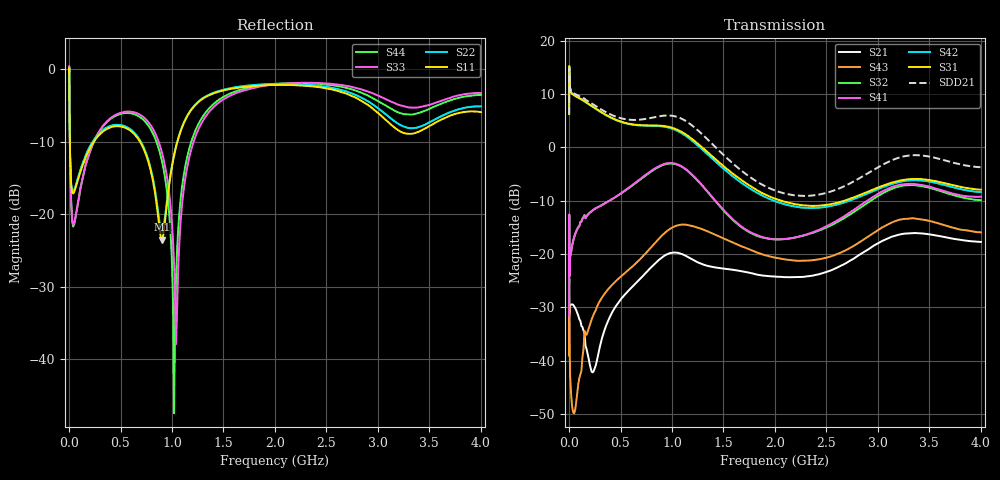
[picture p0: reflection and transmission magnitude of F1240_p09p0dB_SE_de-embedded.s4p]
! Integrated Device Technology
! Corporate Headquarters
! 6024 Silver Creek Valley Road
! San Jose, CA 95138  USA
! Phone:  1-408-284-8200
! Toll Free:  1-800-223-1366
! Webpage:  http://www.idt.com/
! Timing and RF Division
! 515 Groton Road, Suite 102
! Westford, MA 01886-6024
! Device:  F1240
! Description: Dual Intermediate Frequency Digital Variable Gain Amplifier
! Frequency:  10.0 -  500.00 MHz
! Package:  5x5 mm QFN Plastic Package: 32 pin
! Ports:  8 RF, 20 DC
!  Pin  1  = GA3 / Data  Pin 17  = RF OUT_B+
!  Pin  2  = GA4 / CLK  Pin 18  = RF OUT_B-
!  Pin  3  = GA5  Pin 19  = STBY_B
!  Pin  4  = VMODE  Pin 20  = Ground
!  Pin  5  = No Connect  Pin 21  = Ground
!  Pin  6  = GB5  Pin 22  = STB_A
!  Pin  7  = GB4  Pin 23  = RF OUT_A-  = Port 4
!  Pin  8  = GB3  Pin 24  = RF OUT_A+  = Port 3
!  Pin  9  = GB2  Pin 25  = GA0
!  Pin 10  = GB1  Pin 26  = ISET_A
!  Pin 11  = RF IN_B+  Pin 27  = VCC
!  Pin 12  = RF IN_B-  Pin 28  = Ground
!  Pin 13  = Ground  Pin 29  = RF IN_A-  = Port 2
!  Pin 14  = VCC  Pin 30  = RF IN_A+  = Port 1
!  Pin 15  = ISET_B  Pin 31  = GA1
!  Pin 16  = GB0  Pin 32  = GA2 / CSb
! Gain  = +19.5 dB
! State  = 1
! Voltage  = +5.00 V
! Current  = 85.292 mA (one channel only)
! Temperture  =  +25 C
! Test Date  =  2017-10-18
! Board  =  EB4031
! Data:  The device was measured on a custom evaluation board which has
!  individual transmission lines to the RF pins.  Data was collected
!  using a calibrated network analyzer.  The evaluation board was
!  de-embedded using Automatic Fixture Removal.
!  The reference plane is the edge of the package pin.
!  Only Channel A was measured.
!  This data is in single-ended operation.  If your needs are balanced
!  or differential S-parameters then this file needs to be used a
!  linear simulator.
! File Date:  2017-11-10  MJV
! Note:
!  Integrated Device Technology supplies this data as a sample of measured
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# Hz S dB R 100
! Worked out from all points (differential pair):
!   410 points, 500 kHz to 4 GHz, reference 100 ohm
!   strongest paths, dB at 500 kHz, 930 MHz, 1.96 GHz, 2.98 GHz, 4 GHz:
!     S31: 6.2, 4.0, -9.3, -7.7, -8.0
!     S42: 6.2, 3.8, -9.8, -8.0, -8.4
!     S41: -31.7, -3.1, -17.2, -9.0, -9.3
!     S32: -31.3, -3.2, -17.2, -9.4, -9.9
!     S43: -39.0, -16.1, -20.5, -15.8, -15.9
!     S21: -25.5, -20.3, -24.2, -18.2, -17.8
!   taken as a pair (ports 1,2 in; 3,4 out), SDD21 dB: 6.3, 5.9, -7.8, -4.0, -3.7
!   lowest |S11| = -23.5 dB at 900 MHz (marker M1), VSWR 1.14, Z = 111 + j8.88 ohm
!   |S11| at or under -10 dB: 8.138 MHz to 239.6 MHz (231.5 MHz wide, 187 % of centre); 690 MHz to 1.052 GHz (361.8 MHz wide, 41.5 % of centre)
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500000  -0.41 -5.6  -25.52 -4.8  -27.19 81.8  -57.90 69.0
        -25.54 -5.0  -0.41 -5.6  -58.32 68.7  -27.20 83.0
        6.24 -105.1  -31.30 16.1  -0.50 1.4  -39.05 -101.8
        -31.73 13.6  6.22 -103.9  -39.03 -101.4  -0.50 3.7
3000000  -2.83 -59.3  -31.43 -36.9  -15.96 24.8  -56.83 19.2
         -31.42 -36.0  -2.80 -59.3  -56.99 20.2  -15.97 25.0
         14.42 -179.3  -20.50 126.0  -2.32 -54.8  -31.28 162.0
         -20.80 124.1  14.42 -179.1  -31.27 162.1  -2.38 -54.6
2e8  -10.95 -135.6  -40.52 -45.2  -17.94 -50.4  -34.23 19.7
     -40.61 -40.7  -10.69 -136.6  -34.19 20.4  -17.96 -50.5
     8.00 109.7  -12.27 -12.1  -11.45 -99.3  -33.90 111.0
     -12.31 -12.7  7.97 109.0  -33.35 107.7  -11.50 -98.3
5.3e8  -7.97 177.5  -28.42 -12.1  -19.09 -108.8  -28.61 -55.9
       -27.88 -13.8  -7.79 176.4  -28.73 -53.9  -19.21 -109.0
       4.65 26.5  -8.36 -79.2  -5.88 -158.8  -24.63 11.8
       -8.28 -80.7  4.59 25.7  -23.79 10.2  -6.05 -158.8
9e8  -23.51 36.6  -20.87 -85.3  -17.02 171.0  -25.42 -142.9
     -20.69 -91.5  -22.52 37.4  -25.67 -136.4  -17.31 170.4
     4.03 -65.7  -3.44 -179.9  -11.35 136.9  -17.45 -68.2
     -3.30 176.3  3.92 -67.5  -16.61 -71.7  -12.52 137.8
1.21e9  -5.18 -112.6  -20.34 -172.1  -19.07 85.5  -25.29 143.3
        -21.19 -175.9  -5.11 -112.4  -24.92 150.4  -19.68 84.4
        1.32 -157.6  -5.48 70.6  -9.96 -98.8  -15.37 -163.5
        -5.43 65.8  1.00 -159.5  -14.84 -167.0  -9.04 -103.6
4e9  -5.90 -151.2  -17.87 80.0  -20.54 -63.6  -21.03 -47.9
     -17.75 79.3  -5.10 -148.1  -22.41 -28.5  -22.50 -56.4
     -7.96 21.5  -9.92 -97.0  -3.26 -139.2  -16.77 85.0
     -9.27 -110.8  -8.41 29.5  -15.95 60.1  -3.52 -146.3
